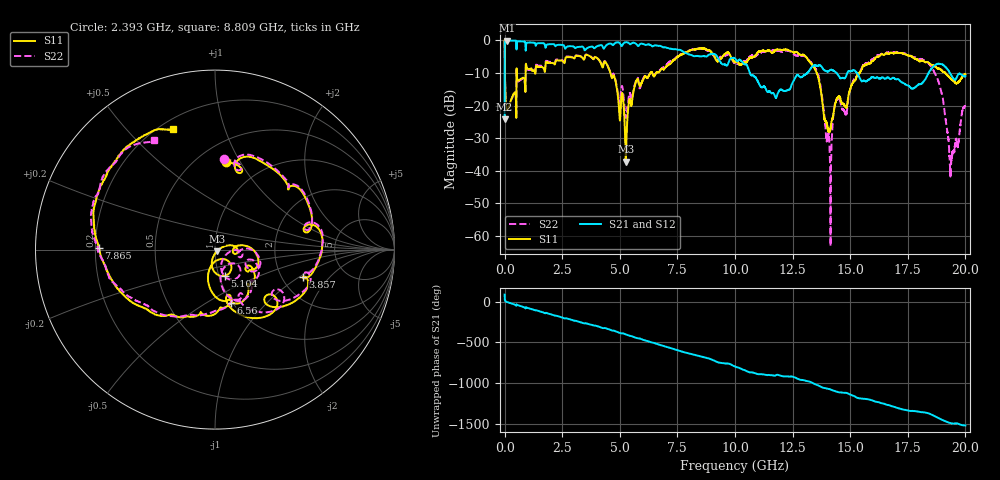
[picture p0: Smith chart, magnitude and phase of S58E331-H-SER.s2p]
!{S58E331}
!Johanson Technology Inc.
!www.johansontechnology.com
!Test Board Conditions:
!Substrate Type  RO4350B
!Substrate Thickness  60 mil
!Substrate Dk  3.66
!TL Type: GCPW
!TL Trace Width  115 mil
!TL Gap  52 mil
!Electrode orientation  Horizontal
!DUT TOPOLOGY	SERIES
!Mounting Pad LxW  55x428 mil
! Created Wed Apr 14 11:43:16 2021
# mhz S ma R 50
! 2 Port Network Data from SP1.SP block
! freq  magS11  angS11  magS21  angS21  magS12  angS12  magS22  angS22
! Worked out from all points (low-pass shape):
!   20001 points, 300 kHz to 20 GHz, reference 50 ohm
!   highest |S21| = -0.09 dB at 95.3 MHz (marker M1); lowest = -24.2 dB at 300 kHz (marker M2)
!   |S21| within 3 dB of the highest: 4.88 MHz to 915.1 MHz (910.2 MHz wide, 198 % of centre); 918.7 MHz to 7.663 GHz (6.745 GHz wide, 157 % of centre)
!   lowest |S11| = -37.2 dB at 5.259 GHz (marker M3), VSWR 1.03, Z = 51 - j0.954 ohm
!   |S11| at or under -10 dB: 4.593 GHz to 6.329 GHz (1.736 GHz wide, 31.8 % of centre); 13.55 GHz to 15.41 GHz (1.865 GHz wide, 12.9 % of centre); 19.13 GHz to end of sweep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
!   |S22| runs from -63.1 to 0.0 dB; largest |S21 - S12| = 0.0088
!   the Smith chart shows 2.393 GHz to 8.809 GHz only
!   S11 on the Smith chart (normalised r, x): 2.393 GHz: 0.67, +0.87; 3.857 GHz: 2.59, -1.08; 5.104 GHz: 1.07, -0.32; 6.56 GHz: 0.99, -0.65; 7.865 GHz: 0.21, +0.01; 8.809 GHz: 0.25, +0.68
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0.3  0.9945 -3.9  0.0619 85.5  0.0613 85.7  0.9961 -3.9
95.3  0.08619 -100.2  0.9892 -5.1  0.9882 -5.0  0.0857 -100.1
1149.3  0.3696 177.6  0.9247 -91.6  0.9245 -91.6  0.3568 179.8
2393.3  0.492 83.2  0.8535 172.8  0.8539 172.8  0.5056 84.3
3334.3  0.5579 14.8  0.8011 103.3  0.8007 103.3  0.5619 15.8
3857.3  0.5124 -17.4  0.7769 65.6  0.7765 65.5  0.5174 -14.3
5104.3  0.1562 -68.9  0.8279 -29.7  0.8271 -29.7  0.1982 -56.6
5259.3  0.01381 -42.6  0.9343 -44.3  0.935 -44.3  0.06623 -39.5
6560.3  0.3101 -73.0  0.8391 -156.2  0.8379 -156.2  0.3131 -74.8
6667.3  0.3268 -83.8  0.8233 -165.8  0.8219 -165.9  0.338 -86.5
7865.3  0.6467 179.0  0.6394 92.4  0.6386 92.3  0.6527 179.6
8809.3  0.7126 109.3  0.5796 25.1  0.5812 25.2  0.6971 119.0
10000.3  0.4606 59.5  0.5293 -79.8  0.5291 -79.8  0.4439 58.5
12104.3  0.7181 -87.3  0.1679 161.3  0.1679 161.6  0.6762 -89.6
13334.3  0.4284 170.3  0.3925 84.5  0.3925 84.6  0.443 174.9
14104.3  0.04003 41.0  0.3458 4.4  0.347 4.1  0.0236 157.3
14418.3  0.1272 -101.5  0.3139 -28.7  0.3125 -28.8  0.1234 -119.5
16667.3  0.6196 58.6  0.2683 167.5  0.2613 167.1  0.6455 60.7
17885.3  0.5122 -67.9  0.1989 91.6  0.1981 91.9  0.5375 -71.3
18573.3  0.4161 179.8  0.3851 44.7  0.3838 44.7  0.3673 178.0
19392.3  0.2523 37.7  0.291 -57.5  0.2938 -58.1  0.01519 -2.8
20000  0.301 -76.0  0.2824 -82.6  0.2826 -82.5  0.09721 -99.3
